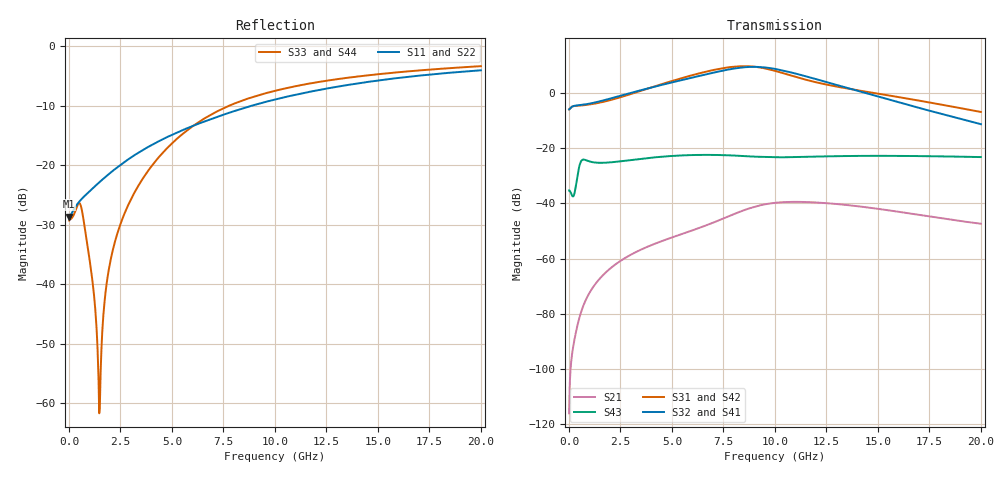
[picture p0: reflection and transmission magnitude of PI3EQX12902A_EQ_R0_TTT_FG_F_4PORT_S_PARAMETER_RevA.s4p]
! NPort=4 DATA=2000 NOISE=0 GROUPDELAY=0 COMPLEX_DATAFORMAT=POLAR
! NumOfBlock=1 NumOfParam=0
! .MODEL Smodel S TSTONEFILE=PI3EQX12902A_EQ_R0_TTT_FG_F_4PORT_S_PARAMETER_RevA.s4p TYPE=S
!  -- The above .MODEL line can be used for the S element in the netlist.
! The s parameter is extracted from the linear redriver, it is not bi-directional; only s(4,1)s(4,2) and s(3,1)s(3,2)
! should be the insertion loss
!Port definition:
!Port1 = input+
!Port2 = input-
!Port3 = output+
!Port4 = output-
# Hz S MA R  50
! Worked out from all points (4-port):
!   2000 points, 10 MHz to 20 GHz, reference 50 ohm
!   strongest paths, dB at 10 MHz, 5.01 GHz, 10.01 GHz, 15.01 GHz, 20 GHz:
!     S32: -6.0, 3.7, 8.6, -1.4, -11.4
!     S41: -6.0, 3.7, 8.6, -1.4, -11.3
!     S31: -6.0, 4.2, 7.9, -0.4, -7.0
!     S42: -6.0, 4.1, 7.7, -0.6, -7.2
!     S43: -35.3, -22.9, -23.4, -22.8, -23.3
!     S21: -116.0, -52.4, -39.8, -42.0, -47.4
!   lowest |S11| = -28.6 dB at 10 MHz (marker M1), VSWR 1.08, Z = 46.4 - j0.0607 ohm
!   |S11| at or under -10 dB: start of sweep to 8.878 GHz
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1e7  0.03704 -179.0  1.588e-06 51.9  0 0.0  0 0.0
     1.588e-06 51.9  0.03704 -179.0  0 0.0  0 0.0
     0.4993 0.9  0.4993 -179.1  0.03429 6.0  0.01709 -177.1
     0.4993 -179.1  0.4993 0.9  0.01709 -177.1  0.03429 6.0
1.49e9  0.07219 -133.4  0.0004305 116.4  3.744e-09 177.2  5.624e-09 -173.9
        0.0004305 116.4  0.07219 -133.4  5.625e-09 -173.8  3.745e-09 177.2
        0.6597 6.2  0.696 -179.4  0.0008858 -60.3  0.05389 -174.9
        0.694 -179.4  0.6595 5.9  0.05389 -174.8  0.0009453 -62.8
6.13e9  0.2176 -112.1  0.003368 86.5  1.857e-06 -26.5  1.127e-06 84.8
        0.003368 86.5  0.2176 -112.1  1.134e-06 85.0  1.852e-06 -26.3
        2.14 -46.8  1.927 107.0  0.2199 -47.9  0.07421 143.2
        1.922 107.0  2.107 -47.3  0.07462 143.3  0.2193 -47.9
9.33e9  0.3331 -113.3  0.009224 46.3  1.202e-05 -125.5  9.126e-06 -7.9
        0.009256 46.3  0.3331 -113.3  9.223e-06 -8.1  1.203e-05 -125.4
        2.831 -143.4  2.898 5.8  0.3925 -76.7  0.06842 114.1
        2.89 6.0  2.784 -143.8  0.06882 113.9  0.3921 -76.6
1.102e10  0.3921 -115.9  0.01055 10.7  1.724e-05 -167.1  1.447e-05 -67.7
          0.01059 10.4  0.3921 -115.9  1.461e-05 -68.0  1.725e-05 -167.0
          1.922 172.8  2.205 -51.4  0.4621 -87.5  0.06821 105.3
          2.201 -51.1  1.883 172.3  0.06842 105.0  0.4621 -87.4
1.355e10  0.4729 -120.2  0.00924 -28.4  2.687e-05 147.4  1.855e-05 -137.1
          0.009242 -28.8  0.4728 -120.2  1.87e-05 -137.4  2.684e-05 147.4
          1.183 133.6  1.206 -114.5  0.5438 -100.0  0.07146 88.5
          1.209 -114.1  1.151 133.5  0.07145 88.2  0.5442 -99.9
2e10  0.6271 -131.5  0.004341 -71.4  4.396e-05 50.1  1.759e-05 105.6
      0.004264 -71.5  0.6272 -131.5  1.775e-05 105.0  4.387e-05 50.2
      0.4477 44.5  0.2692 136.3  0.6794 -119.6  0.06847 46.2
      0.272 136.3  0.4385 45.1  0.0684 46.1  0.6797 -119.6
